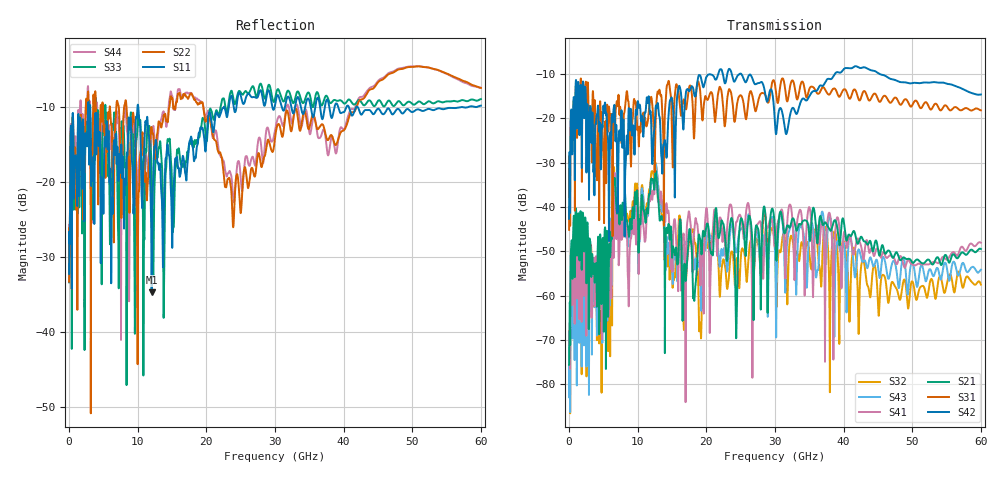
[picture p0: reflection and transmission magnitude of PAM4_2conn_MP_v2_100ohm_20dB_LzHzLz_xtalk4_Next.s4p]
! Info: Touchstone file created by Circ.  Input file=FAB50GbE_2conn_Midplane_Examax_Topo2_v2_100ohm_20dB_LzHzLz.circ
# Hz S RI R 50
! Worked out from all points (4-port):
!   6000 points, 10 MHz to 60 GHz, reference 50 ohm
!   strongest paths, dB at 10 MHz, 15.01 GHz, 30.01 GHz, 45.01 GHz, 60 GHz:
!     S42: -42.6, -15.7, -21.2, -9.7, -14.6
!     S31: -45.1, -24.9, -12.4, -15.7, -18.2
!     S21: -75.6, -51.4, -45.6, -49.5, -49.4
!     S41: -68.0, -52.1, -48.6, -49.5, -48.0
!     S43: -71.0, -53.0, -50.3, -53.3, -54.1
!     S32: -74.8, -54.6, -50.1, -61.9, -57.5
!   lowest |S11| = -34.7 dB at 12.03 GHz (marker M1), VSWR 1.04, Z = 51.1 - j1.52 ohm
!   |S11| at or under -10 dB: 3.086 GHz to 9.965 GHz (6.879 GHz wide, 105 % of centre); 10.09 GHz to 22.52 GHz (12.43 GHz wide, 76.2 % of centre); 42.08 GHz to 56.91 GHz (14.83 GHz wide, 30 % of centre)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
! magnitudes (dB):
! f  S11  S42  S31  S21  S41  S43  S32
! 10 MHz  -32.2  -42.6  -45.1  -75.6  -68.0  -71.0  -74.8
! 1.17 GHz  -22.5  -21.7  -24.4  -50.2  -53.8  -57.9  -55.7
! 12.03 GHz  -34.7  -25.5  -15.5  -33.6  -37.4  -34.1  -31.9
! 19.11 GHz  -12.8  -10.3  -13.9  -47.3  -55.8  -55.6  -66.2
! 19.88 GHz  -15.9  -11.3  -14.9  -45.4  -42.0  -49.4  -46.8
! 28.48 GHz  -9.8  -13.6  -14.4  -40.1  -47.8  -46.2  -41.0
! 60 GHz  -9.8  -14.6  -18.2  -49.4  -48.0  -54.1  -57.5
